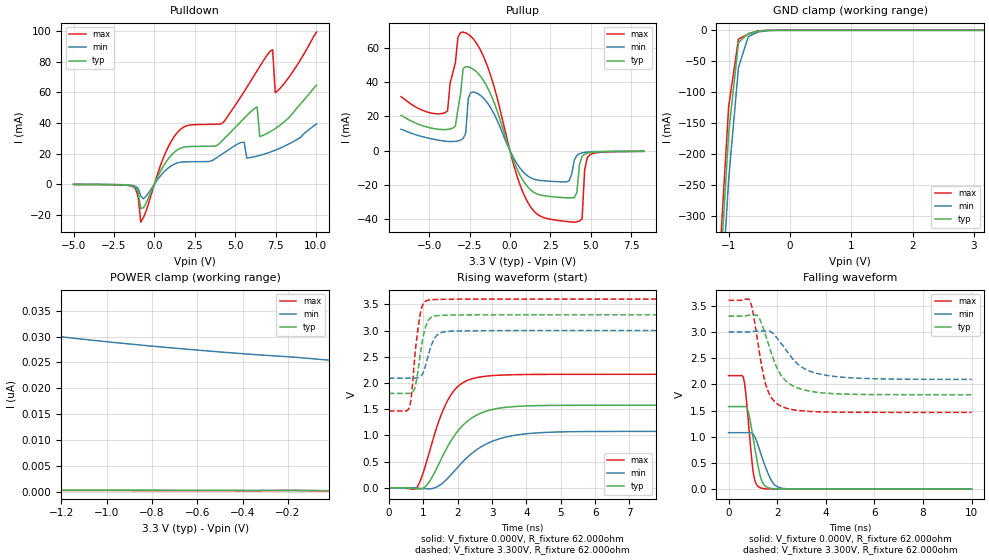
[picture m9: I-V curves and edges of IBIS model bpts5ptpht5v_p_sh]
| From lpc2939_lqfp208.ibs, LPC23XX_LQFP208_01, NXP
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| |   Rev 0.20 IBIS Model Design Automation Generation   |
| |   N O N - S I L I C O N   C O R R E L A T E D   |
| |   This IBIS [Model] is pre-Beta tactical support   |
| |  Note: this IBIS [Model] contains clamp curves generated   |
| |   through simulation which should not be relied upon   |
| Pccmos14 hliolib_nlm 4.0.1
|   0.18 um 3.3V pad library
|   six level metal
|   dual oxide
|   single threshold voltage
|   nominal line mixed supply
|   parasitic extracted netlists
| Process block c14
| bpts5ptpht5v
|   Bidirectional Pad 3v3
|   3state Output
|   Plain Input
|   1ns Slew Rate control
|   CMOS
|   Programmable between
|   - (p1=0, p2=1) plain input
|   - (p1=0, p2=0) with Pull Up
|   - (p1=1, p2=1) with Pull Down
|   - (p1=1, p2=0) with Repeater
|   Characterized at Core 1.8V and I/O 3.3V
| Plain input Mode (p1=0, p2=1)
[Model]   bpts5ptpht5v_p_sh | of bpts5ptpht5v
Model_type   I/O
Polarity   Non-Inverting
Enable   Active-Low
|  Reciever Thresholds
Vinl   = 0.99V
Vinh   = 2.31V
| AC Test Load Conditions
Vref   = 0
Cref   = 1.2e-11
Rref   = 1000000000
Vmeas   = 1.65
| [Process Range]   typical   min   max
| C_comp edge width   400.000ps   400.000ps   400.000ps
| C_comp Tstrobe   40.000fs   40.000fs   40.000fs
C_comp   2.522pF   2.389pF   2.658pF
[Temperature Range]   25   125   -40
[Voltage Range]   3.30V   3.00V   3.60V
[GND Clamp Reference]   0.00V   0.00V   0.00V
[Pulldown Reference]   0.00V   0.00V   0.00V
[POWER Clamp Reference]   3.30V   3.00V   3.60V
[Pullup Reference]   3.30V   3.00V   3.60V
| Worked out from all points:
|   slope of the pulldown table from 0 to 0.495 V, typ, clamps not added: 46.5 ohm
|   slope of the pullup table from 0 to 0.495 V, typ, clamps not added: 41.9 ohm
|   GND clamp passes 1 mA (typ) near -0.49 V on its own axis
|   rising waveform, V_fixture 0.000V, R_fixture 62.000ohm: 20-80 % time 919ps typ, 1.16ns min, 699ps max; typ from 0 V to 1.57 V
|   falling waveform, V_fixture 0.000V, R_fixture 62.000ohm: 20-80 % time 364ps typ, 510ps min, 256ps max; typ from 1.57 V to 0 V
|   rising waveform, V_fixture 3.300V, R_fixture 62.000ohm: 20-80 % time 223ps typ, 262ps min, 202ps max; typ from 1.8 V to 3.3 V
|   falling waveform, V_fixture 3.300V, R_fixture 62.000ohm: 20-80 % time 811ps typ, 1.12ns min, 530ps max; typ from 3.3 V to 1.8 V
[GND Clamp]
| ref voltage   0.00V   0.00V   0.00V
|   Voltage   I(typ)   I(min)   I(max)
-5V       -7.933A    -7.953A    -7.929A
-1.16V    -429.6mA   -501mA     -389.4mA
-1V       -166mA     -240.8mA   -123.1mA
-840mV    -19.69mA   -60.07mA   -14.09mA
-680mV    -5.152mA   -10.14mA   -6.089mA
-520mV    -1.268mA   -2.624mA   -791.9uA
-200mV    -120.2nA   -8.927uA   -2.485nA
3.16V     214.9pA    26.04nA    149.6pA
[Power Clamp]   | Vtable = Vcc - Vpad
| ref voltage   3.30V   3.00V   3.60V
|   Voltage   I(typ)   I(min)   I(max)
-6.74V    1.25nA     125.5nA    594.5pA
-4.66V    766.7pA    70.58nA    463.5pA
-2.42V    452.4pA    38.32nA    329.5pA
-2.26V    435.5pA    36.92nA    320pA
-2.1V     419.2pA    35.63nA    310.6pA
-1.78V    388.2pA    33.31nA    291.8pA
-1.62V    373.4pA    32.29nA    282.4pA
-1.3V     345pA      30.47nA    263.6pA
-980mV    318.1pA    28.92nA    244.8pA
-660mV    292.5pA    27.62nA    226.1pA
-180mV    257pA      26.06nA    260.4pA
-20mV     229.7pA    25.46nA    172.4pA
[Pulldown]
| ref voltage   0.00V   0.00V   0.00V
|   Voltage   I(typ)   I(min)   I(max)
-5V       -187.5uA   -145.7uA   -211.8uA
-1.32V    -1.32mA    -939.3uA   -1.723mA
-1V       -5.321mA   -2.96mA    -8.615mA
-840mV    -15.95mA   -7.733mA   -24.9mA
1.4V      22.26mA    13.79mA    33.48mA
4.28V     29.27mA    20.27mA    40.55mA
5.56V     43.15mA    27.33mA    60.63mA
6.36V     50.49mA    18.36mA    74.24mA
6.52V     31.16mA    18.79mA    76.97mA
7.32V     35.27mA    21.55mA    87.95mA
7.48V     36.36mA    22.22mA    59.78mA
10.04V    64.68mA    39.32mA    99.49mA
[Pullup]   | Vtable = Vcc - Vpad
| ref voltage   3.30V   3.00V   3.60V
|   Voltage   I(typ)   I(min)   I(max)
-6.74V    20.65mA    12.57mA    31.52mA
-3.86V    12.45mA    5.473mA    23.29mA
-3.22V    24.39mA    5.73mA     66.13mA
-2.9V     47.88mA    7.139mA    69.22mA
-2.42V    48.4mA     34.05mA    66.69mA
780mV     -16.88mA   -11.92mA   -23.75mA
2.38V     -26.56mA   -17.72mA   -39.71mA
3.98V     -27.38mA   -5.508mA   -41.66mA
4.46V     -3.36mA    -1.235mA   -39.9mA
4.62V     -2.02mA    -961.4uA   -11.27mA
4.94V     -1.105mA   -662.2uA   -2.417mA
8.3V      -310.5uA   -276uA     -365.2uA
[Ramp]
R_load   = 62.000ohm
|   dV/dt(typ)   dV/dt(min)   dV/dt(max)
dV/dt_r   723.230mV/915.000ps   485.705mV/1.125ns   1.051V/765.000ps
dV/dt_f   678.874mV/810.000ps   404.697mV/1.100ns   1.041V/590.000ps
[Rising Waveform]  | cubic spline decimation from 2001 points
V_fixture   = 0.000V
R_fixture   = 62.000ohm
|   Time   V(typ)   V(min)   V(max)
0s        2.056nV    364.8nV    1.069nV
820ps     -20.79mV   -5.721mV   13.81mV
1.15ns    91.69mV    -19.91mV   616.8mV
1.395ns   377mV      16.23mV    1.159V
1.635ns   695.3mV    131.7mV    1.568V
1.97ns    1.053V     367.8mV    1.909V
2.35ns    1.303V     620.6mV    2.066V
3.05ns    1.499V     897.5mV    2.142V
4.03ns    1.562V     1.033V     2.161V
10ns      1.575V     1.077V     2.165V
[Falling Waveform]  | cubic spline decimation from 2001 points
V_fixture   = 0.000V
R_fixture   = 62.000ohm
|   Time   V(typ)   V(min)   V(max)
0s        1.575V     1.077V     2.165V
610ps     1.576V     1.077V     2.124V
795ps     1.498V     1.078V     1.396V
1.01ns    978.3mV    1.051V     342mV
1.12ns    679mV      957.6mV    119.6mV
1.29ns    276.8mV    728.7mV    30.22mV
1.47ns    78.04mV    484.9mV    9.766mV
1.775ns   11.72mV    154.2mV    2.851mV
2.22ns    2.488mV    16.51mV    1.172mV
10ns      416.5nV    6.231uV    21.32nV
[Rising Waveform]  | cubic spline decimation from 2001 points
V_fixture   = 3.300V
V_fixture_min = 3.000V
V_fixture_max = 3.600V
R_fixture   = 62.000ohm
|   Time   V(typ)   V(min)   V(max)
0s        1.8V       2.092V     1.464V
600ps     1.801V     2.093V     1.546V
650ps     1.809V     2.092V     1.725V
765ps     1.926V     2.092V     2.583V
895ps     2.464V     2.116V     3.25V
980ps     2.825V     2.176V     3.482V
1.12ns    3.159V     2.463V     3.576V
1.35ns    3.279V     2.873V     3.591V
1.705ns   3.293V     2.983V     3.596V
10ns      3.3V       3V         3.6V
[Falling Waveform]  | cubic spline decimation from 2001 points
V_fixture   = 3.300V
V_fixture_min = 3.000V
V_fixture_max = 3.600V
R_fixture   = 62.000ohm
|   Time   V(typ)   V(min)   V(max)
0s        3.3V       3V         3.6V
880ps     3.318V     3.001V     3.59V
995ps     3.32V      3.006V     3.396V
1.19ns    3.309V     3.014V     2.842V
1.52ns    2.94V      3.014V     2.012V
1.82ns    2.516V     2.973V     1.709V
2.2ns     2.148V     2.759V     1.574V
2.935ns   1.917V     2.352V     1.498V
3.965ns   1.832V     2.175V     1.472V
10ns      1.8V       2.093V     1.464V
